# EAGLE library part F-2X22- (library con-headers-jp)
FEMALE HEADER
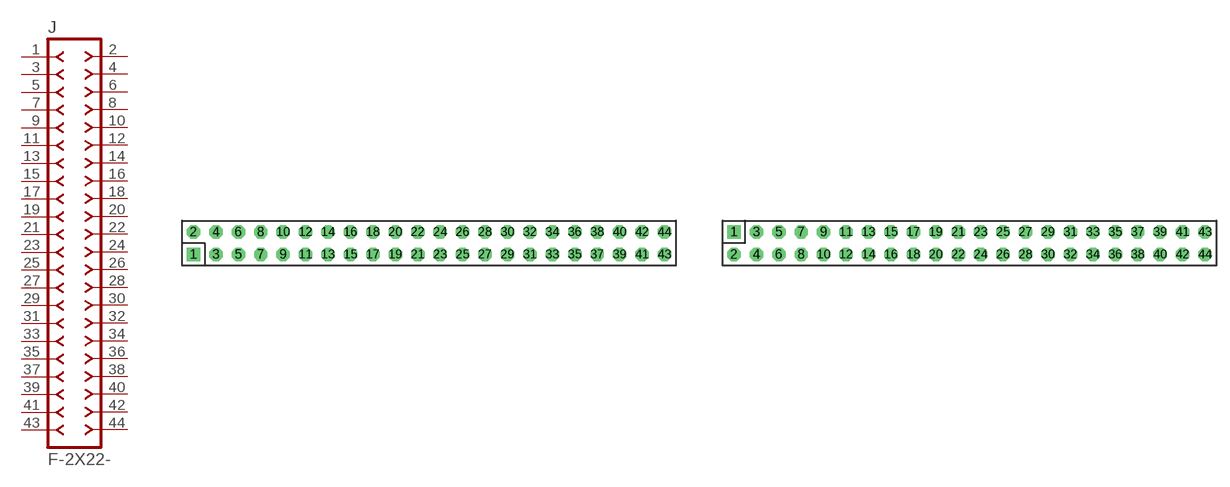
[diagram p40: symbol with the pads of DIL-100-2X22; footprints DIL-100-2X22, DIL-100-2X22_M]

Designator prefix J

## F-2X22-DIL-100  [DIL-100-2X22]
1  1  pas
2  2  pas
3  3  pas
4  4  pas
5  5  pas
6  6  pas
7  7  pas
8  8  pas
9  9  pas
10  10  pas
11  11  pas
12  12  pas
13  13  pas
14  14  pas
15  15  pas
16  16  pas
17  17  pas
18  18  pas
19  19  pas
20  20  pas
21  21  pas
22  22  pas
23  23  pas
24  24  pas
25  25  pas
26  26  pas
27  27  pas
28  28  pas
29  29  pas
30  30  pas
31  31  pas
32  32  pas
33  33  pas
34  34  pas
35  35  pas
36  36  pas
37  37  pas
38  38  pas
39  39  pas
40  40  pas
41  41  pas
42  42  pas
43  43  pas
44  44  pas

## F-2X22-DIL-100_M  [DIL-100-2X22_M]
Pads as for DIL-100-2X22

## F-2X22-DIL-2MM  [DIL-2MM-2X22]
Pads as for DIL-100-2X22

## F-2X22-DIL-2MM_M  [DIL-2MM-2X22_M]
Pads as for DIL-100-2X22

## Footprint DIL-100-2X22 (pad centres in mm)
PIN HEADER - 0.1"
drill 1.016 square: 1 -26.67,-1.27
drill 1.016 octagon: 2 -26.67,1.27; 3 -24.13,-1.27; 4 -24.13,1.27; 5 -21.59,-1.27; 6 -21.59,1.27; 7 -19.05,-1.27; 8 -19.05,1.27; 9 -16.51,-1.27; 10 -16.51,1.27; 11 -13.97,-1.27; 12 -13.97,1.27; 13 -11.43,-1.27; 14 -11.43,1.27; 15 -8.89,-1.27; 16 -8.89,1.27; 17 -6.35,-1.27; 18 -6.35,1.27; 19 -3.81,-1.27; 20 -3.81,1.27; 21 -1.27,-1.27; 22 -1.27,1.27; 23 1.27,-1.27; 24 1.27,1.27; 25 3.81,-1.27; 26 3.81,1.27; 27 6.35,-1.27; 28 6.35,1.27; 29 8.89,-1.27; 30 8.89,1.27; 31 11.43,-1.27; 32 11.43,1.27; 33 13.97,-1.27; 34 13.97,1.27; 35 16.51,-1.27; 36 16.51,1.27; 37 19.05,-1.27; 38 19.05,1.27; 39 21.59,-1.27; 40 21.59,1.27; 41 24.13,-1.27; 42 24.13,1.27; 43 26.67,-1.27; 44 26.67,1.27

## Footprint DIL-100-2X22_M (pad centres in mm)
PIN HEADER - MIRRORED 0.1"
drill 1.016 square: 1 -26.67,1.27
drill 1.016 octagon: 2 -26.67,-1.27; 3 -24.13,1.27; 4 -24.13,-1.27; 5 -21.59,1.27; 6 -21.59,-1.27; 7 -19.05,1.27; 8 -19.05,-1.27; 9 -16.51,1.27; 10 -16.51,-1.27; 11 -13.97,1.27; 12 -13.97,-1.27; 13 -11.43,1.27; 14 -11.43,-1.27; 15 -8.89,1.27; 16 -8.89,-1.27; 17 -6.35,1.27; 18 -6.35,-1.27; 19 -3.81,1.27; 20 -3.81,-1.27; 21 -1.27,1.27; 22 -1.27,-1.27; 23 1.27,1.27; 24 1.27,-1.27; 25 3.81,1.27; 26 3.81,-1.27; 27 6.35,1.27; 28 6.35,-1.27; 29 8.89,1.27; 30 8.89,-1.27; 31 11.43,1.27; 32 11.43,-1.27; 33 13.97,1.27; 34 13.97,-1.27; 35 16.51,1.27; 36 16.51,-1.27; 37 19.05,1.27; 38 19.05,-1.27; 39 21.59,1.27; 40 21.59,-1.27; 41 24.13,1.27; 42 24.13,-1.27; 43 26.67,1.27; 44 26.67,-1.27

## Footprint DIL-2MM-2X22 (pad centres in mm)
PIN HEADER - 2MM
drill 0.711 square: 1 -21,-1
drill 0.711: 2 -21,1; 3 -19,-1; 4 -19,1; 5 -17,-1; 6 -17,1; 7 -15,-1; 8 -15,1; 9 -13,-1; 10 -13,1; 11 -11,-1; 12 -11,1; 13 -9,-1; 14 -9,1; 15 -7,-1; 16 -7,1; 17 -5,-1; 18 -5,1; 19 -3,-1; 20 -3,1; 21 -1,-1; 22 -1,1; 23 1,-1; 24 1,1; 25 3,-1; 26 3,1; 27 5,-1; 28 5,1; 29 7,-1; 30 7,1; 31 9,-1; 32 9,1; 33 11,1; 34 11,-1; 35 13,1; 36 13,-1; 37 15,1; 38 15,-1; 39 17,1; 40 17,-1; 41 19,-1; 42 19,1; 43 21,-1; 44 21,1

## Footprint DIL-2MM-2X22_M (pad centres in mm)
PIN HEADER - MIRRORED 2MM
drill 0.711 square: 1 -21,1
drill 0.711: 2 -21,-1; 3 -19,1; 4 -19,-1; 5 -17,1; 6 -17,-1; 7 -15,1; 8 -15,-1; 9 -13,1; 10 -13,-1; 11 -11,1; 12 -11,-1; 13 -9,1; 14 -9,-1; 15 -7,1; 16 -7,-1; 17 -5,1; 18 -5,-1; 19 -3,1; 20 -3,-1; 21 -1,1; 22 -1,-1; 23 1,1; 24 1,-1; 25 3,1; 26 3,-1; 27 5,1; 28 5,-1; 29 7,1; 30 7,-1; 31 9,1; 32 9,-1; 33 11,-1; 34 11,1; 35 13,-1; 36 13,1; 37 15,-1; 38 15,1; 39 17,-1; 40 17,1; 41 19,1; 42 19,-1; 43 21,1; 44 21,-1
